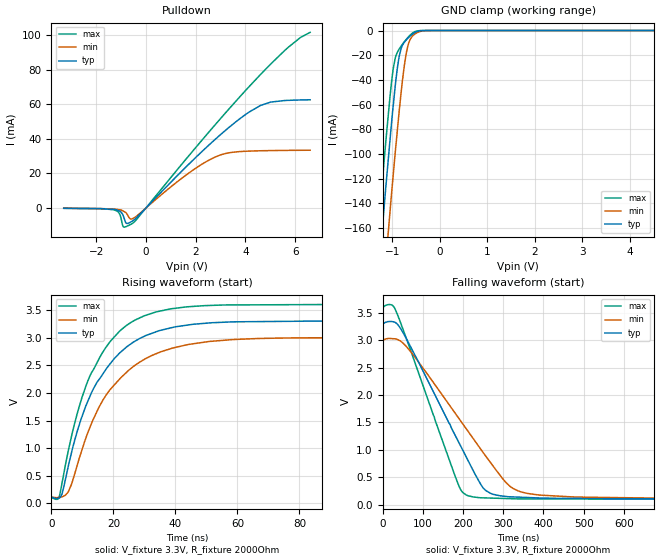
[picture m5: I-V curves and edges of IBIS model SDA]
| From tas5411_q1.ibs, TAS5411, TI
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|   Model
[Model]   SDA
Model_type   I/O_open_drain
Polarity   Non-Inverting
Enable   Active-Low
Vinl = 0.9
Vinh = 2.13
Vmeas = 1.65
Vref = 3.3
Cref = 1pF
Rref = 2000
|   typ   min   max
C_comp   1.316pF   1.269pF   1.523pF
[Voltage Range]   3.3   3   3.6
[Temperature Range]   27   125   -40
[Pullup Reference]   3.3   3   3.6
[Pulldown Reference]   0   0   0
[Power Clamp Reference]   3.3   3   3.6
[GND Clamp Reference]   0   0   0
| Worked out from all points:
|   slope of the pulldown table from 0 to 0.495 V, typ, clamps not added: 66.6 ohm
|   GND clamp passes 1 mA (typ) near -0.49 V on its own axis
|   falling waveform, V_fixture 3.3V, R_fixture 2000Ohm: 20-80 % time 132ns typ, 169ns min, 101ns max; typ from 3.3 V to 0.106 V
|   rising waveform, V_fixture 3.3V, R_fixture 2000Ohm: 20-80 % time 15.2ns typ, 16.9ns min, 13.7ns max; typ from 0.106 V to 3.3 V
[Pulldown]
|   Voltage   I(typ)   I(min)   I(max)
-3.3V     -131.3uA   -128.2uA   -128.1uA
-1.3V     -762.6uA   -568.1uA   -961.8uA
-1.092V   -1.507mA   -933.7uA   -2.524mA
-904.2mV  -4.576mA   -1.803mA   -10.85mA
-765.6mV  -8.924mA   -3.292mA   -10.53mA
-627mV    -8.217mA   -6.256mA   -9.579mA
-528mV    -7.402mA   -6.108mA   -8.776mA
1.68V     24.74mA    19.77mA    29.46mA
2.927V    41.57mA    30.34mA    50.56mA
4.61V     59.38mA    33.14mA    77.34mA
5.719V    62.3mA     33.37mA    92.98mA
6.6V      62.64mA    33.45mA    101.6mA
[GND Clamp]
|   Voltage   I(typ)   I(min)   I(max)
-3.3V     -1.18A     -1.236A    -1.145A
-1.29V    -198.8mA   -258.8mA   -161.1mA
-1.241V   -175.8mA   -235.7mA   -138.1mA
-1.162V   -139.7mA   -199.7mA   -102.3mA
-1.132V   -126.2mA   -186.2mA   -89.21mA
-1.041V   -86.77mA   -144.8mA   -51.76mA
-973.5mV  -59.28mA   -115.2mA   -29.99mA
-854.7mV  -21.46mA   -66.24mA   -15.13mA
-765.6mV  -10.7mA    -34.83mA   -10.2mA
-696.3mV  -7.304mA   -17.06mA   -6.83mA
-518.1mV  -1.551mA   -2.742mA   -849.3uA
6.6V      0A         0A         0A
[POWER Clamp]
|   Voltage   I(typ)   I(min)   I(max)
-3.3V     0A         0A         0A
2.977V    0A         0A         0A
3.066V    0A         0A         0A
6.6V      0A         0A         0A
[Ramp]
R_load = 2000
|   typ   min   max
dV/dt_r   1.91615/1.52423e-08   1.73027/1.68812e-08   2.10032/1.36734e-08
dV/dt_f   1.91614/1.31447e-07   1.73026/1.68782e-07   2.10032/1.01081e-07
[Falling Waveform]
V_fixture = 3.3V
V_fixture_min = 3V
V_fixture_max = 3.6V
R_fixture = 2000Ohm
C_fixture = 0F
|   Time   V(typ)   V(min)   V(max)
0s        3.3V       3V         3.6V
22ns      3.34V      3.028V     3.643V
33.75ns   3.309V     3.02V      3.521V
74.5ns    2.808V     2.745V     2.711V
180.2ns   1.267V     1.67V      521.1mV
208.1ns   867.9mV    1.383V     177.9mV
257.2ns   255.6mV    878.4mV    124.9mV
306.4ns   152.2mV    407.5mV    114.1mV
351.2ns   135.5mV    221.6mV    107.7mV
1us       106.4mV    116.1mV    99.46mV
[Rising Waveform]
V_fixture = 3.3V
V_fixture_min = 3V
V_fixture_max = 3.6V
R_fixture = 2000Ohm
C_fixture = 0F
|   Time   V(typ)   V(min)   V(max)
0s        106.4mV    116mV      99.46mV
2.63ns    101.4mV    112.1mV    141.3mV
3.42ns    170mV      119.6mV    366.2mV
5.388ns   659mV      202.4mV    936.7mV
11.12ns   1.766V     1.185V     2.125V
15.28ns   2.237V     1.736V     2.608V
18.89ns   2.523V     2.057V     2.926V
30.29ns   3.034V     2.617V     3.402V
49.34ns   3.259V     2.918V     3.579V
1us       3.3V       3V         3.6V
